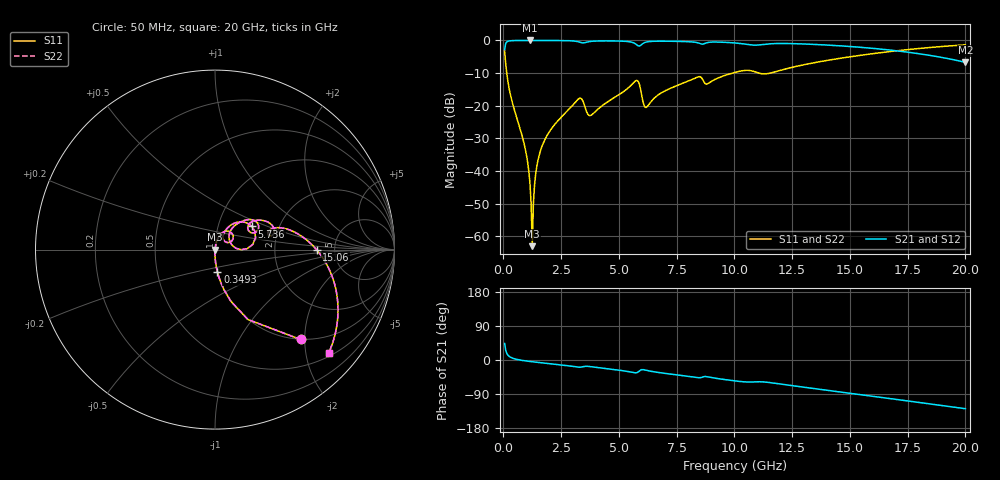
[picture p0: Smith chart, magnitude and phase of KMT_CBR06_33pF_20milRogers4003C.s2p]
! Data measured by Modelithics Inc. support@modelithics.com 813-866-6335
! KEMET CBR0603 33pF, Pad Width= 0.851mm, Pad Length= 0.64mm, Pad Gap= 0.62mm, 20mil Rogers 4003C substrate Data, January 2022
# hz S ma R 50
! 2 Port Network Data from SP1.SP block
! freq  magS11  angS11  magS21  angS21  magS12  angS12  magS22  angS22
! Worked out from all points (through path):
!   401 points, 50 MHz to 20 GHz, reference 50 ohm
!   highest |S21| = -0.01 dB at 1.147 GHz (marker M1); lowest = -6.7 dB at 20 GHz (marker M2)
!   group delay of S21, straight-line fit = 18 ps
!   lowest |S11| = -63.0 dB at 1.247 GHz (marker M3), VSWR 1.00, Z = 50.1 + j0.000906 ohm
!   |S11| at or under -10 dB: 142.8 MHz to 9.914 GHz (9.771 GHz wide, 194 % of centre); 11.06 GHz to 11.55 GHz (490 MHz wide, 4.33 % of centre)
!   |S22| runs from -63.0 to -1.4 dB; largest |S21 - S12| = 0
!   S11 on the Smith chart (normalised r, x): 50 MHz: 0.99, -1.91; 349.2 MHz: 1.00, -0.25; 5.736 GHz: 1.45, +0.40; 15.06 GHz: 3.61, -0.00; 20 GHz: 0.57, -2.47
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5e7  0.6913 -46.4  0.7222 43.5  0.7222 43.5  0.6913 -46.4
1.99625e8  0.2279 -77.5  0.9733 12.4  0.9733 12.4  0.2279 -77.5
3.4925e8  0.1256 -83.9  0.9917 5.9  0.9917 5.9  0.1256 -83.9
9.4775e8  0.0216 -90.7  0.9991 -2.3  0.9991 -2.3  0.0216 -90.7
1.0475e9  0.01365 -90.4  0.9992 -3.1  0.9992 -3.1  0.01365 -90.4
1.14725e9  0.006521 -87.9  0.9993 -3.9  0.9993 -3.9  0.006521 -87.9
1.247e9  0.0007103 0.7  0.9992 -4.6  0.9992 -4.6  0.0007103 0.7
1.34675e9  0.006211 77.8  0.9992 -5.3  0.9992 -5.3  0.006211 77.8
1.496375e9  0.01472 80.5  0.999 -6.4  0.999 -6.4  0.01472 80.5
1.795625e9  0.03042 79.8  0.9985 -8.4  0.9985 -8.4  0.03042 79.8
3.391625e9  0.1266 36.5  0.9218 -18.4  0.9218 -18.4  0.1266 36.5
3.790625e9  0.07165 47.4  0.9676 -17.7  0.9676 -17.7  0.07165 47.4
5.73575e9  0.2423 32.2  0.8764 -33.8  0.8764 -33.8  0.2423 32.2
6.184625e9  0.09455 29.6  0.9449 -27.2  0.9449 -27.2  0.09455 29.6
6.73325e9  0.1493 51.2  0.974 -33.2  0.974 -33.2  0.1493 51.2
8.379125e9  0.2732 36.3  0.9267 -46.2  0.9267 -46.2  0.2732 36.3
8.828e9  0.2161 32.2  0.9269 -44.2  0.9269 -44.2  0.2161 32.2
1.0025e10  0.3242 29.2  0.9143 -55.2  0.9143 -55.2  0.3242 29.2
1.336662e10  0.4502 12.8  0.8721 -74.6  0.8721 -74.6  0.4502 12.8
1.506238e10  0.5657 -0.0  0.8049 -88.1  0.8049 -88.1  0.5657 -0.0
1.670825e10  0.6742 -13.5  0.714 -101.5  0.714 -101.5  0.6742 -13.5
2e10  0.856 -42.3  0.4627 -128.5  0.4627 -128.5  0.856 -42.3
